| IBIS file stm32mp211_213_215_vfbga273.ibs
[IBIS ver] 5.1
[File name] stm32mp211_213_215_vfbga273.ibs
[File Rev] 0.4
[Date] 09-10-2025
[Source] Data Created at STMicroelectronics
[Notes]  File originated from ELDO simulations.
[Disclaimer]  This information is for modeling purpose only and is
   not guaranted. The information is subject to change without
   notice.
[Copyright] Copyright 2025 STMicroelectronics Inc.
|   Component stm32mp211_213_215_vfbga273
[Component] stm32mp211_213_215_vfbga273
[Manufacturer] STMicroelectronics
[Package]
| variable   typ   min   max
R_pkg  0  NA  NA
L_pkg  0  NA  NA
C_pkg  0  NA  NA
[Pin]   signal_name   model_name
1A1  VSS  gnd
1A3  VSS  gnd
1A5  VSS  gnd
1A7  VSS  gnd
1B2  VSS  gnd
1B4  VSS  gnd
1B6  VDDCPU  nc
1B8  VSS  gnd
1C1  VDDCORE  nc
1C3  VDDCORE  nc
1C5  VDDCPU  nc
1C7  VDDCPU  nc
1D2  VDDCORE  nc
1D4  VDDCORE  nc
1D6  VDDCPU  nc
1D8  VDDCPU  nc
1E1  VSS  gnd
1E3  VSS  gnd
1E5  VSS  gnd
1E7  VSS  gnd
1F2  VSS  gnd
1F4  VSS  gnd
1F6  VSS  gnd
1F8  VSS  gnd
1G1  VDD  power
1G3  VDD  power
1G5  VDDCORE  nc
1G7  VSS  gnd
1H2  VDD  power
1H4  VDD  power
1H6  VDDCORE  nc
1H8  VDDCORE  nc
A1  VSS  gnd
A2  CSI_D1P  DPHY_IBIS_L1
A3  CSI_CKP  DPHY_IBIS_L1
A6  PD3  io8_tt
A7  PD15  io8_tt_i3c
A10  PB1  io8_tt
A11  PE0  io8_tt
A14  PE13  io8_tt
A15  PE12  io8_tt
A18  PB12  io8_tt
A19  PD13  io8_tt
A20  DDR_DQ11  mal4drv27_PAD
A21  VSS  gnd
AA1  VSS  gnd
AA2  OSC_OUT  isudq_v18
AA3  BOOT2  isudq_tt
AA6  PF10  io8_tt
AA7  PF9  io8_tt
AA10  PA14  io8_tt
AA11  PF2  io8_tt_i3c
AA14  PH12  io8_tt
AA15  PH7  io8_tt
AA18  PH4  io8_tt
AA19  USBH_HS_DM  USB2_HS_IBIS
AA20  OTG_TXRTUNE  nc
AA21  VSS  gnd
B1  CSI_D0P  DPHY_IBIS_L1
B2  CSI_D1N  DPHY_IBIS_L1
B3  CSI_CKN  DPHY_IBIS_L1
B4  PD10  io8_tt_i3c
B6  PD4  io8_tt
B7  PD8  io8_tt
B8  PB9  io8_tt
B10  PB3  io8_tt
B11  PD6  io8_tt
B12  PE2  io8_tt
B14  PE11  io8_tt
B15  PE9  io8_tt
B16  PB14  io8_tt
B18  PD12  io8_tt
B19  DDR_DQ10  mal4drv27_PAD
B20  DDR_DQ9  mal4drv27_PAD
B21  DDR_DQ8  mal4drv27_PAD
C1  CSI_D0N  DPHY_IBIS_L1
C2  VDDCSI  nc
C3  CSI_REXT  nc
C4  PD2  io8_tt
C5  PB7  io8_tt
C6  PB11  io8_tt
C7  PD1  io8_tt
C8  PB10  io8_tt
C9  PD9  io8_tt
C10  PD5  io8_tt
C11  PE1  io8_tt
C12  PE3  io8_tt
C13  PE8  io8_tt
C14  PE7  io8_tt
C15  PE10  io8_tt
C16  PB13  io8_tt
C17  PD14  io8_tt
C18  DDR_RESETN  nc
C19  DDR_DQ15  mal4drv27_PAD
C20  DDR_DQS1N  mal4drv27_PAD
C21  DDR_DQS1P  mal4drv27_PAD
D2  VDDA18CSI  power
D3  PI6  io8_tt
D4  PD11  io8_tt_i3c
D6  PB6  io8_tt
D8  PD0  io8_tt
D10  PE5  io8_tt
D12  PE4  io8_tt
D14  PE14  io8_tt
D16  VDDA18PLL1  nc
D18  DDR_A9  mal4drv20_PAD
D19  DDR_DQ14  mal4drv27_PAD
D20  DDR_DQM1  mal4drv27_PAD
E3  PG2  io8_tt_i3c
E4  PC5  io8_tt_i3c
E5  PI5  io8_tt
E7  PB5  io8_tt_i3c
E9  PB2  io8_tt
E11  PE15  io8_tt
E13  PE6  io8_tt
E15  PD7  io8_tt
E17  DDR_A3  mal4drv20_PAD
E19  DDR_DQ12  mal4drv27_PAD
F1  PI1  io8_tt_i3c
F2  PA7  io8_tt
F3  PF5  io8_tt
F4  PI0  io8_tt
F6  VSS  gnd
F8  VDDIO3  power
F10  VDDIO3  power
F12  VDDIO2  power
F14  VDDIO1  power
F16  VDDA18DDR  nc
F18  DDR_A20  mal4drv20_PAD
F19  DDR_DQ13  mal4drv27_PAD
F20  DDR_A11  mal4drv20_PAD
F21  DDR_A21  mal4drv20_PAD
G1  PG14  io8_tt
G2  PG15  io8_tt
G3  PF6  io8_tt
G5  PI4  io8_tt
G17  DDR_A0  mal4drv20_PAD
G19  DDR_A1  mal4drv20_PAD
G20  DDR_A10  mal4drv20_PAD
G21  DDR_A22  mal4drv20_PAD
H2  PG12  io8_tt
H3  PG11  io8_tt
H4  PG10  io8_tt
H6  V08CAP  nc
H16  VDDQDDR  power
H18  DDR_A25  mal4drv20_PAD
H19  DDR_A8  mal4drv20_PAD
H20  DDR_A23  mal4drv20_PAD
J3  PG9  io8_tt
J5  PC0  io8_tt
J17  DDR_A18  mal4drv20_PAD
J19  DDR_A2  mal4drv20_PAD
K1  PA5  io8_tt
K2  PH5  io8_tt
K3  PG8  io8_tt
K4  PZ0  io8_tt_i3c_tamp
K6  PZ3  io8_tt_i3c_tamp
K16  VDDQDDR  power
K18  DDR_A31  mal4drv20_PAD
K19  DDR_A14  mal4drv20_PAD
K20  DDR_A26  mal4drv20_PAD
K21  DDR_A13  mal4drv20_PAD
L1  VDDA18AON  power
L2  VSSAON  nc
L3  PG7  io8_tt
L5  PZ1  io8_tt_i3c_tamp
L17  DDR_A12  mal4drv20_PAD
L19  DDR_A27  mal4drv20_PAD
L20  DDR_A5  mal4drv20_PAD
L21  DDR_A4  mal4drv20_PAD
M2  PA10  io8_tt
M3  PF4  io8_tt
M4  PG5  io8_tt
M6  VBAT  power
M16  VDDQDDR  power
M18  DDR_A6  mal4drv20_PAD
M19  DDR_A28  mal4drv20_PAD
M20  DDR_A15  mal4drv20_PAD
N3  PB15  io8_tt
N5  PA1  io8_tt_i3c
N17  DDR_ZQ  nc
N19  DDR_A16  mal4drv20_PAD
P1  PF13  io8_tt
P2  PF15  io8_tt
P3  PC11  io8_tt
P4  PF7  io8_tt
P6  PG4  io8_tt
P16  VDDQDDR  power
P18  DDR_A7  mal4drv20_PAD
P19  DDR_A29  mal4drv20_PAD
P20  DDR_A17  mal4drv20_PAD
P21  DDR_A30  mal4drv20_PAD
R1  OSC32_IN  isudq_v18
R2  OSC32_OUT  isudq_v18
R3  PDR_ON  nc
R5  PC4  io8_tt
R17  VDDA18PLL2  nc
R19  DDR_DQ6  mal4drv27_PAD
R20  DDR_DQ4  mal4drv27_PAD
R21  DDR_DQ5  mal4drv27_PAD
T2  NRSTC1MS  io8_tt
T3  PG13  io8_tt_i3c
T4  PC13  io8_tt
T6  VSSA  nc
T8  PG0  io8_tt_i3c
T10  PC7  io8_tt
T12  PC3  io8_tt
T14  PF8  io8_tt
T16  PA9  io8_tt
T18  DDR_VREF  nc
T19  DDR_DQS0P  mal4drv27_PAD
T20  DDR_DQ7  mal4drv27_PAD
U3  PF12  io8_tt
U5  PI8  io8_tt
U7  PG1  io8_tt_i3c
U9  PC10  io8_tt
U11  PA15  io8_tt_i3c
U13  PF3  io8_tt
U15  PH9  io8_tt
U17  DDR_DQM0  mal4drv27_PAD
U19  DDR_DQS0N  mal4drv27_PAD
V1  JTCK_SWCLK  io8_tt
V2  JTMS_SWDIO  io8_tt
V3  NJTRST  io8_tt
V4  PWR_CPUON  io8_tt
V6  PG3  io8_tt
V8  ANA0  nc
V10  PC1  io8_tt_i3c
V12  PA13  io8_tt
V14  PH10  io8_tt
V16  PA8  io8_tt_i3c
V18  VDDA18USB  power
V19  DDR_DQ1  mal4drv27_PAD
V20  DDR_DQ0  mal4drv27_PAD
V21  DDR_DQ2  mal4drv27_PAD
W1  JTDO_TRACESWO  io8_tt
W2  JTDI  io8_tt
W3  PWR_LP  io8_tt
W4  PWR_ON  io8_tt
W5  BOOT3  isudq_tt
W6  VDDA18ADC  power
W7  PF11  io8_tt
W8  VREFN  nc
W9  ANA1  nc
W10  PC9  io8_tt
W11  PF1  io8_tt
W12  PC6  io8_tt_i3c
W13  PH13  io8_tt
W14  PH11  io8_tt
W15  PA11  io8_tt
W16  PA6  io8_tt
W17  PA2  io8_tt_i3c
W18  VSS  gnd
W19  VDD33USB  power
W20  USBH_HS_TXRTUNE  nc
W21  DDR_DQ3  mal4drv27_PAD
Y1  NRST  nc
Y2  OSC_IN  isudq_v18
Y3  BOOT1  isudq_tt
Y4  BOOT0  isudq_tt
Y6  PA0  io8_tt
Y7  PC12  io8_tt_i3c
Y8  VREFP  nc
Y10  PC8  io8_tt
Y11  PF0  io8_tt_i3c
Y12  PC2  io8_tt
Y14  PA12  io8_tt_i3c
Y15  PH8  io8_tt
Y16  PA4  io8_tt
Y18  PA3  io8_tt_i3c
Y19  USBH_HS_DP  USB2_HS_IBIS
Y20  OTG_HSDP  USB2_HS_IBIS
Y21  OTG_HSDM  USB2_HS_IBIS
[Package Model]   503-fcvfbga-11x11-273-240814
[Pin Mapping]   pulldown_ref   pullup_ref   | Comment
1A1  gnd  nc
1A3  gnd  nc
1A5  gnd  nc
1A7  gnd  nc
1B2  gnd  nc
1B4  gnd  nc
1B6  nc  nc
1B8  gnd  nc
1C1  nc  nc
1C3  nc  nc
1C5  nc  nc
1C7  nc  nc
1D2  nc  nc
1D4  nc  nc
1D6  nc  nc
1D8  nc  nc
1E1  gnd  nc
1E3  gnd  nc
1E5  gnd  nc
1E7  gnd  nc
1F2  gnd  nc
1F4  gnd  nc
1F6  gnd  nc
1F8  gnd  nc
1G1  nc  vdd
1G3  nc  vdd
1G5  nc  nc
1G7  gnd  nc
1H2  nc  vdd
1H4  nc  vdd
1H6  nc  nc
1H8  nc  nc
A1  gnd  nc
A2  gnd  VDDA18CSI
A3  gnd  VDDA18CSI
A6  gnd  vddio3
A7  gnd  vdd
A10  gnd  vdd
A11  gnd  vddio1
A14  gnd  vddio2
A15  gnd  vddio2
A18  gnd  vdd
A19  gnd  vdd
A20  gnd  vddqddr
A21  gnd  nc
AA1  gnd  nc
AA2  gnd  vdda18aon
AA3  gnd  vdd
AA6  gnd  vdd
AA7  gnd  vdd
AA10  gnd  vdd
AA11  gnd  vdd
AA14  gnd  vdd
AA15  gnd  vdd
AA18  gnd  vdd
AA19  gnd  VDD33USB
AA20  nc  nc
AA21  gnd  nc
B1  gnd  VDDA18CSI
B2  gnd  VDDA18CSI
B3  gnd  VDDA18CSI
B4  gnd  vddio3
B6  gnd  vddio3
B7  gnd  vddio3
B8  gnd  vdd
B10  gnd  vdd
B11  gnd  vddio3
B12  gnd  vddio1
B14  gnd  vddio2
B15  gnd  vddio1
B16  gnd  vdd
B18  gnd  vdd
B19  gnd  vddqddr
B20  gnd  vddqddr
B21  gnd  vddqddr
C1  gnd  VDDA18CSI
C2  nc  nc
C3  nc  nc
C4  gnd  vddio3
C5  gnd  vdd
C6  gnd  vdd
C7  gnd  vddio3
C8  gnd  vdd
C9  gnd  vddio3
C10  gnd  vddio3
C11  gnd  vddio1
C12  gnd  vddio1
C13  gnd  vddio1
C14  gnd  vddio1
C15  gnd  vddio2
C16  gnd  vdd
C17  gnd  vdd
C18  nc  nc
C19  gnd  vddqddr
C20  gnd  vddqddr
C21  gnd  vddqddr
D2  nc  VDDA18CSI
D3  gnd  vdd
D4  gnd  vddio3
D6  gnd  vdd
D8  gnd  vddio3
D10  gnd  vddio1
D12  gnd  vddio1
D14  gnd  vddio2
D16  nc  nc
D18  gnd  vddqddr
D19  gnd  vddqddr
D20  gnd  vddqddr
E3  gnd  vdd
E4  gnd  vdd
E5  gnd  vdd
E7  gnd  vdd
E9  gnd  vdd
E11  gnd  vddio2
E13  gnd  vddio1
E15  gnd  vddio3
E17  gnd  vddqddr
E19  gnd  vddqddr
F1  gnd  vdd
F2  gnd  vdd
F3  gnd  vdd
F4  gnd  vdd
F6  gnd  nc
F8  nc  vddio3
F10  nc  vddio3
F12  nc  vddio2
F14  nc  vddio1
F16  nc  nc
F18  gnd  vddqddr
F19  gnd  vddqddr
F20  gnd  vddqddr
F21  gnd  vddqddr
G1  gnd  vdd
G2  gnd  vdd
G3  gnd  vdd
G5  gnd  vdd
G17  gnd  vddqddr
G19  gnd  vddqddr
G20  gnd  vddqddr
G21  gnd  vddqddr
H2  gnd  vdd
H3  gnd  vdd
H4  gnd  vdd
H6  nc  nc
H16  nc  vddqddr
H18  gnd  vddqddr
H19  gnd  vddqddr
H20  gnd  vddqddr
J3  gnd  vdd
J5  gnd  vdd
J17  gnd  vddqddr
J19  gnd  vddqddr
K1  gnd  vdd
K2  gnd  vdd
K3  gnd  vdd
K4  gnd  vdd  | Depending on IO usage
| K4  gnd  vsw  | Depending on IO usage
K6  gnd  vdd  | Depending on IO usage
| K6  gnd  vsw  | Depending on IO usage
K16  nc  vddqddr
K18  gnd  vddqddr
K19  gnd  vddqddr
K20  gnd  vddqddr
K21  gnd  vddqddr
L1  nc  vdda18aon
L2  nc  nc
L3  gnd  vdd
L5  gnd  vdd  | Depending on IO usage
| L5  gnd  vsw  | Depending on IO usage
L17  gnd  vddqddr
L19  gnd  vddqddr
L20  gnd  vddqddr
L21  gnd  vddqddr
M2  gnd  vdd
M3  gnd  vdd
M4  gnd  vdd
M6  nc  vsw
M16  nc  vddqddr
M18  gnd  vddqddr
M19  gnd  vddqddr
M20  gnd  vddqddr
N3  gnd  vdd
N5  gnd  vdd
N17  nc  nc
N19  gnd  vddqddr
P1  gnd  vdd
P2  gnd  vdd
P3  gnd  vdd
P4  gnd  vdd
P6  gnd  vdd
P16  nc  vddqddr
P18  gnd  vddqddr
P19  gnd  vddqddr
P20  gnd  vddqddr
P21  gnd  vddqddr
R1  gnd  vdd  | Depending on IO usage
| R1  gnd  vsw  | Depending on IO usage
R2  gnd  vdd  | Depending on IO usage
| R2  gnd  vsw  | Depending on IO usage
R3  nc  nc
R5  gnd  vdd
R17  nc  nc
R19  gnd  vddqddr
R20  gnd  vddqddr
R21  gnd  vddqddr
T2  gnd  vdd
T3  gnd  vdd
T4  gnd  vdd  | Depending on IO usage
| T4  gnd  vsw  | Depending on IO usage
T6  nc  nc
T8  gnd  vdd
T10  gnd  vdd
T12  gnd  vdd
T14  gnd  vdd
T16  gnd  vdd
T18  nc  nc
T19  gnd  vddqddr
T20  gnd  vddqddr
U3  gnd  vdd
U5  gnd  vdd
U7  gnd  vdd
U9  gnd  vdd
U11  gnd  vdd
U13  gnd  vdd
U15  gnd  vdd
U17  gnd  vddqddr
U19  gnd  vddqddr
V1  gnd  vdd
V2  gnd  vdd
V3  gnd  vdd
V4  gnd  vdd
V6  gnd  vdd
V8  nc  nc
V10  gnd  vdd
V12  gnd  vdd
V14  gnd  vdd
V16  gnd  vdd
V18  nc  vdda18usb
V19  gnd  vddqddr
V20  gnd  vddqddr
V21  gnd  vddqddr
W1  gnd  vdd
W2  gnd  vdd
W3  gnd  vdd
W4  gnd  vdd
W5  gnd  vdd
W6  nc  vdda18adc
W7  gnd  vdd
W8  nc  nc
W9  nc  nc
W10  gnd  vdd
W11  gnd  vdd
W12  gnd  vdd
W13  gnd  vdd
W14  gnd  vdd
W15  gnd  vdd
W16  gnd  vdd
W17  gnd  vdd
W18  gnd  nc
W19  nc  VDD33USB
W20  nc  nc
W21  gnd  vddqddr
Y1  nc  nc
Y2  gnd  vdda18aon
Y3  gnd  vdd
Y4  gnd  vdd
Y6  gnd  vdd
Y7  gnd  vdd
Y8  nc  nc
Y10  gnd  vdd
Y11  gnd  vdd
Y12  gnd  vdd
Y14  gnd  vdd
Y15  gnd  vdd
Y16  gnd  vdd
Y18  gnd  vdd
Y19  gnd  VDD33USB
Y20  gnd  VDD33USB
Y21  gnd  VDD33USB
[Diff Pin]  inv_pin  vdiff  tdelay_typ  tdelay_min  tdelay_max
B3  A3  NA  NA  NA  NA
C1  B1  NA  NA  NA  NA
B2  A2  NA  NA  NA  NA
T19  U19  NA  NA  NA  NA
C21  C20  NA  NA  NA  NA
Y19  AA19  NA  NA  NA  NA   |USBH_HS_DP _DM
Y20  Y21  NA  NA  NA  NA   |USBH_HS_DP _DM
L21  L20  NA  NA  NA  NA
[Model Selector] USB2_HS_IBIS
USB2_HSRX   USB2 HSRX model
USB2_HSTX_00_0_01_0011_11   TuningBits_AMP_PULSE_RISE_REF_XV=00_0_01_0011_11
USB2_HSTX_00_0_10_0101_11   TuningBits_AMP_PULSE_RISE_REF_XV=00_0_10_0101_11
USB2_HSTX_00_0_11_0111_11   TuningBits_AMP_PULSE_RISE_REF_XV=00_0_11_0111_11
USB2_HSTX_00_1_01_0011_11   TuningBits_AMP_PULSE_RISE_REF_XV=00_1_01_0011_11
USB2_HSTX_00_1_10_0101_11   TuningBits_AMP_PULSE_RISE_REF_XV=00_1_10_0101_11
USB2_HSTX_00_1_11_0111_11   TuningBits_AMP_PULSE_RISE_REF_XV=00_1_11_0111_11
USB2_HSTX_01_0_01_0011_11   TuningBits_AMP_PULSE_RISE_REF_XV=01_0_01_0011_11
USB2_HSTX_01_0_10_0101_11   TuningBits_AMP_PULSE_RISE_REF_XV=01_0_10_0101_11
USB2_HSTX_01_0_11_0111_11   TuningBits_AMP_PULSE_RISE_REF_XV=01_0_11_0111_11
USB2_HSTX_01_1_01_0011_11   TuningBits_AMP_PULSE_RISE_REF_XV=01_1_01_0011_11
USB2_HSTX_01_1_10_0101_11   TuningBits_AMP_PULSE_RISE_REF_XV=01_1_10_0101_11
USB2_HSTX_01_1_11_0111_11   TuningBits_AMP_PULSE_RISE_REF_XV=01_1_11_0111_11
USB2_HSTX_10_0_01_0011_11   TuningBits_AMP_PULSE_RISE_REF_XV=10_0_01_0011_11
USB2_HSTX_10_0_10_0101_11   TuningBits_AMP_PULSE_RISE_REF_XV=10_0_10_0101_11
USB2_HSTX_10_0_11_0111_11   TuningBits_AMP_PULSE_RISE_REF_XV=10_0_11_0111_11
USB2_HSTX_10_1_01_0011_11   TuningBits_AMP_PULSE_RISE_REF_XV=10_1_01_0011_11
USB2_HSTX_10_1_10_0101_11   TuningBits_AMP_PULSE_RISE_REF_XV=10_1_10_0101_11
USB2_HSTX_10_1_11_0111_11   TuningBits_AMP_PULSE_RISE_REF_XV=10_1_11_0111_11
[Model Selector] DPHY_IBIS_L1
DPHY_RX_2P5G_L1   DPHY HSRX model at 2.5Gbps for lane 1
DPHY_RX_1P5G_L1   DPHY HSRX model at 1.5Gbps for lane 1
[Model Selector] io8_tt
io8_tt_ls_3v3 "GPIO - 3V tolerant - low speed - 3.3V range"
io8_tt_ms_3v3 "GPIO - 3V tolerant - med speed - 3.3V range"
io8_tt_fs_3v3 "GPIO - 3V tolerant - fast speed - 3.3V range"
io8_tt_hs_3v3 "GPIO - 3V tolerant - high speed - 3.3V range"
io8_tt_hslv_ls_1v8 "GPIO low voltage optimization - 3V tolerant - low speed - 1.8V range"
io8_tt_hslv_ms_1v8 "GPIO low voltage optimization - 3V tolerant - med speed - 1.8V range"
io8_tt_hslv_fs_1v8 "GPIO low voltage optimization - 3V tolerant - fast speed - 1.8V range"
io8_tt_hslv_hs_1v8 "GPIO low voltage optimization - 3V tolerant - high speed - 1.8V range"
[Model Selector] io8_tt_i3c
io8_tt_ls_3v3 "GPIO - 3V tolerant - low speed - 3.3V range"
io8_tt_ms_3v3 "GPIO - 3V tolerant - med speed - 3.3V range"
io8_tt_fs_3v3 "GPIO - 3V tolerant - fast speed - 3.3V range"
io8_tt_hs_3v3 "GPIO - 3V tolerant - high speed - 3.3V range"
io8_tt_hslv_ls_1v8 "GPIO low voltage optimization - 3V tolerant - low speed - 1.8V range"
io8_tt_hslv_ms_1v8 "GPIO low voltage optimization - 3V tolerant - med speed - 1.8V range"
io8_tt_hslv_fs_1v8 "GPIO low voltage optimization - 3V tolerant - fast speed - 1.8V range"
io8_tt_hslv_hs_1v8 "GPIO low voltage optimization - 3V tolerant - high speed - 1.8V range"
io8_tt_i3c_ls_3v3 "GPIO with I3C open-drain - 3V tolerant - low speed - 3.3V range"
io8_tt_i3c_ms_3v3 "GPIO with I3C open-drain - 3V tolerant - med speed - 3.3V range"
io8_tt_i3c_fs_3v3 "GPIO with I3C open-drain - 3V tolerant - fast speed - 3.3V range"
io8_tt_i3c_hs_3v3 "GPIO with I3C open-drain - 3V tolerant - high speed - 3.3V range"
io8_tt_hslv_i3c_ls_1v8 "GPIO low voltage optimization with I3C open-drain - 3V tolerant - low speed - 1.8V range"
io8_tt_hslv_i3c_ms_1v8 "GPIO low voltage optimization with I3C open-drain - 3V tolerant - med speed - 1.8V range"
io8_tt_hslv_i3c_fs_1v8 "GPIO low voltage optimization with I3C open-drain - 3V tolerant - fast speed - 1.8V range"
io8_tt_hslv_i3c_hs_1v8 "GPIO low voltage optimization with I3C open-drain - 3V tolerant - high speed - 1.8V range"
io8_tt_i3c_fmp_3v3 "GPIO with I3C fm+ open-drain - 3V tolerant - 3.3V range"
[Model Selector] io8_tt_i3c_tamp
io8_tt_ls_3v3 "GPIO - 3V tolerant - low speed - 3.3V range"
io8_tt_ms_3v3 "GPIO - 3V tolerant - med speed - 3.3V range"
io8_tt_fs_3v3 "GPIO - 3V tolerant - fast speed - 3.3V range"
io8_tt_hs_3v3 "GPIO - 3V tolerant - high speed - 3.3V range"
io8_tt_hslv_ls_1v8 "GPIO low voltage optimization - 3V tolerant - low speed - 1.8V range"
io8_tt_hslv_ms_1v8 "GPIO low voltage optimization - 3V tolerant - med speed - 1.8V range"
io8_tt_hslv_fs_1v8 "GPIO low voltage optimization - 3V tolerant - fast speed - 1.8V range"
io8_tt_hslv_hs_1v8 "GPIO low voltage optimization - 3V tolerant - high speed - 1.8V range"
io8_tt_i3c_ls_3v3 "GPIO with I3C open-drain - 3V tolerant - low speed - 3.3V range"
io8_tt_i3c_ms_3v3 "GPIO with I3C open-drain - 3V tolerant - med speed - 3.3V range"
io8_tt_i3c_fs_3v3 "GPIO with I3C open-drain - 3V tolerant - fast speed - 3.3V range"
io8_tt_i3c_hs_3v3 "GPIO with I3C open-drain - 3V tolerant - high speed - 3.3V range"
io8_tt_hslv_i3c_ls_1v8 "GPIO low voltage optimization with I3C open-drain - 3V tolerant - low speed - 1.8V range"
io8_tt_hslv_i3c_ms_1v8 "GPIO low voltage optimization with I3C open-drain - 3V tolerant - med speed - 1.8V range"
io8_tt_hslv_i3c_fs_1v8 "GPIO low voltage optimization with I3C open-drain - 3V tolerant - fast speed - 1.8V range"
io8_tt_hslv_i3c_hs_1v8 "GPIO low voltage optimization with I3C open-drain - 3V tolerant - high speed - 1.8V range"
io8_tt_i3c_fmp_3v3 "GPIO with I3C fm+ open-drain - 3V tolerant - 3.3V range"
io8_tt_tamp_3v3 "IO tamper - 3V tolerant - 3.3V range"
io8_tt_tamp_1v8 "IO tamper - 3V tolerant - 1.8V range"
[Model Selector] isudq_tt
isudq_tt_3v3 "Input Buffer - 3V tolerant - 3.3V range"
isudq_tt_1v8 "Input Buffer - 3V tolerant - 1.8V range"
|[Model Selector] isudq_v18
|isudq_v18_1v8 "Input Buffer - 1.8V range "
[Model Selector]   mal4drv20_PAD
mal4drv20_d3l_40   DDR3L mal4drv20 cell  Z0=40-Ohm Driver
mal4drv20_d3l_60   DDR3L mal4drv20 cell  Z0=60-Ohm Driver
mal4drv20_d3l_120   DDR3L mal4drv20 cell  Z0=120-Ohm Driver
mal4drv20_d3_20   DDR3 mal4drv20 cell  Z0=20-Ohm Driver
mal4drv20_d3_24   DDR3 mal4drv20 cell  Z0=24-Ohm Driver
mal4drv20_d3_30   DDR3 mal4drv20 cell  Z0=30-Ohm Driver
mal4drv20_d3_40   DDR3 mal4drv20 cell  Z0=40-Ohm Driver
mal4drv20_d3_60   DDR3 mal4drv20 cell  Z0=60-Ohm Driver
mal4drv20_d4_20   DDR4 mal4drv20 cell  Z0=20-Ohm Driver
mal4drv20_d4_24   DDR4 mal4drv20 cell  Z0=24-Ohm Driver
mal4drv20_d4_30   DDR4 mal4drv20 cell  Z0=30-Ohm Driver
mal4drv20_d4_40   DDR4 mal4drv20 cell  Z0=40-Ohm Driver
mal4drv20_d4_60   DDR4 mal4drv20 cell  Z0=60-Ohm Driver
mal4drv20_dl4_20   LPDDR4 mal4drv20 cell  Z0=20-Ohm Driver
mal4drv20_dl4_24   LPDDR4 mal4drv20 cell  Z0=24-Ohm Driver
mal4drv20_dl4_30   LPDDR4 mal4drv20 cell  Z0=30-Ohm Driver
mal4drv20_dl4_40   LPDDR4 mal4drv20 cell  Z0=40-Ohm Driver
mal4drv20_dl4_60   LPDDR4 mal4drv20 cell  Z0=60-Ohm Driver
[Model Selector]   mal4drv27_PAD
mal4drv27_d3l_40   DDR3L mal4drv27 cell  Z0=40-Ohm Driver
mal4drv27_d3l_48   DDR3L mal4drv27 cell  Z0=48-Ohm Driver
mal4drv27_d3l_60   DDR3L mal4drv27 cell  Z0=60-Ohm Driver
mal4drv27_d3l_80   DDR3L mal4drv27 cell  Z0=80-Ohm Driver
mal4drv27_d3l_120   DDR3L mal4drv27 cell  Z0=120-Ohm Driver
mal4drv27_d3l_240   DDR3L mal4drv27 cell  Z0=240-Ohm Driver
mal4drv27_d3l_odt120   DDR3L mal4drv27 cell 120-Ohm ODT Receiver
mal4drv27_d3l_odt60   DDR3L mal4drv27 cell 60-Ohm ODT Receiver
mal4drv27_d3l_odtoff   DDR3L mal4drv27 cell ODT OFF Receiver
mal4drv27_d3_28   DDR3 mal4drv27 cell  Z0=28-Ohm Driver
mal4drv27_d3_34   DDR3 mal4drv27 cell  Z0=34-Ohm Driver
mal4drv27_d3_40   DDR3 mal4drv27 cell  Z0=40-Ohm Driver
mal4drv27_d3_53   DDR3 mal4drv27 cell  Z0=53-Ohm Driver
mal4drv27_d3_odt120   DDR3 mal4drv27 cell 120-Ohm ODT Receiver
mal4drv27_d3_odt60   DDR3 mal4drv27 cell 60-Ohm ODT Receiver
mal4drv27_d4_28   DDR4 mal4drv27 cell  Z0=28-Ohm Driver
mal4drv27_d4_34   DDR4 mal4drv27 cell  Z0=34-Ohm Driver
mal4drv27_d4_40   DDR4 mal4drv27 cell  Z0=40-Ohm Driver
mal4drv27_d4_53   DDR4 mal4drv27 cell  Z0=53-Ohm Driver
mal4drv27_d4_odt120   DDR4 mal4drv27 cell 120-Ohm ODT Receiver
mal4drv27_d4_odt240   DDR4 mal4drv27 cell 240-Ohm ODT Receiver
mal4drv27_d4_odt48   DDR4 mal4drv27 cell 48-Ohm ODT Receiver
mal4drv27_d4_odt60   DDR4 mal4drv27 cell 60-Ohm ODT Receiver
mal4drv27_d4_odt80   DDR4 mal4drv27 cell 80-Ohm ODT Receiver
mal4drv27_dl4_28   LPDDR4 mal4drv27 cell  Z0=28-Ohm Driver
mal4drv27_dl4_34   LPDDR4 mal4drv27 cell  Z0=34-Ohm Driver
mal4drv27_dl4_40   LPDDR4 mal4drv27 cell  Z0=40-Ohm Driver
mal4drv27_dl4_53   LPDDR4 mal4drv27 cell  Z0=53-Ohm Driver
mal4drv27_dl4_odt48   LPDDR4 mal4drv27 cell 48-Ohm ODT Receiver
mal4drv27_dl4_odt60   LPDDR4 mal4drv27 cell 60-Ohm ODT Receiver
[Define Package Model]  503-fcvfbga-11x11-273-240814
[Manufacturer]  unknown
[OEM]  unknown
[Description]  unknown
[Number Of Pins]  235
[Pin Numbers]
| Pin Name Terminal   Net Name   Starting Node   Ending Node
V8 | ANA0
W9 | ANA1
Y4 | BOOT0
Y3 | BOOT1
AA3 | BOOT2
W5 | BOOT3
B3 | CSI_CKN
A3 | CSI_CKP
C1 | CSI_D0N
B1 | CSI_D0P
B2 | CSI_D1N
A2 | CSI_D1P
C3 | CSI_REXT
G17 | DDR_A0
G19 | DDR_A1
J19 | DDR_A2
E17 | DDR_A3
L21 | DDR_A4
L20 | DDR_A5
M18 | DDR_A6
P18 | DDR_A7
H19 | DDR_A8
D18 | DDR_A9
G20 | DDR_A10
F20 | DDR_A11
L17 | DDR_A12
K21 | DDR_A13
K19 | DDR_A14
M20 | DDR_A15
N19 | DDR_A16
P20 | DDR_A17
J17 | DDR_A18
F18 | DDR_A20
F21 | DDR_A21
G21 | DDR_A22
H20 | DDR_A23
H18 | DDR_A25
K20 | DDR_A26
L19 | DDR_A27
M19 | DDR_A28
P19 | DDR_A29
P21 | DDR_A30
K18 | DDR_A31
V20 | DDR_DQ0
V19 | DDR_DQ1
V21 | DDR_DQ2
W21 | DDR_DQ3
R20 | DDR_DQ4
R21 | DDR_DQ5
R19 | DDR_DQ6
T20 | DDR_DQ7
B21 | DDR_DQ8
B20 | DDR_DQ9
B19 | DDR_DQ10
A20 | DDR_DQ11
E19 | DDR_DQ12
F19 | DDR_DQ13
D19 | DDR_DQ14
C19 | DDR_DQ15
U17 | DDR_DQM0
D20 | DDR_DQM1
U19 | DDR_DQS0N
T19 | DDR_DQS0P
C20 | DDR_DQS1N
C21 | DDR_DQS1P
C18 | DDR_RESETN
T18 | DDR_VREF
N17 | DDR_ZQ
V1 | JTCK_SWCLK
W2 | JTDI
W1 | JTDO_TRACESWO
V2 | JTMS_SWDIO
V3 | NJTRST
Y1 | NRST
T2 | NRSTC1MS
R1 | OSC32_IN
R2 | OSC32_OUT
Y2 | OSC_IN
AA2 | OSC_OUT
Y21 | OTG_HSDM
Y20 | OTG_HSDP
AA20 | OTG_TXRTUNE
Y6 | PA0
N5 | PA1
W17 | PA2
Y18 | PA3
Y16 | PA4
K1 | PA5
W16 | PA6
F2 | PA7
V16 | PA8
T16 | PA9
M2 | PA10
W15 | PA11
Y14 | PA12
V12 | PA13
AA10 | PA14
U11 | PA15
A10 | PB1
E9 | PB2
B10 | PB3
E7 | PB5
D6 | PB6
C5 | PB7
B8 | PB9
C8 | PB10
C6 | PB11
A18 | PB12
C16 | PB13
B16 | PB14
N3 | PB15
J5 | PC0
V10 | PC1
Y12 | PC2
T12 | PC3
R5 | PC4
E4 | PC5
W12 | PC6
T10 | PC7
Y10 | PC8
W10 | PC9
U9 | PC10
P3 | PC11
Y7 | PC12
T4 | PC13
D8 | PD0
C7 | PD1
C4 | PD2
A6 | PD3
B6 | PD4
C10 | PD5
B11 | PD6
E15 | PD7
B7 | PD8
C9 | PD9
B4 | PD10
D4 | PD11
B18 | PD12
A19 | PD13
C17 | PD14
A7 | PD15
R3 | PDR_ON
A11 | PE0
C11 | PE1
B12 | PE2
C12 | PE3
D12 | PE4
D10 | PE5
E13 | PE6
C14 | PE7
C13 | PE8
B15 | PE9
C15 | PE10
B14 | PE11
A15 | PE12
A14 | PE13
D14 | PE14
E11 | PE15
Y11 | PF0
W11 | PF1
AA11 | PF2
U13 | PF3
M3 | PF4
F3 | PF5
G3 | PF6
P4 | PF7
T14 | PF8
AA7 | PF9
AA6 | PF10
W7 | PF11
U3 | PF12
P1 | PF13
P2 | PF15
T8 | PG0
U7 | PG1
E3 | PG2
V6 | PG3
P6 | PG4
M4 | PG5
L3 | PG7
K3 | PG8
J3 | PG9
H4 | PG10
H3 | PG11
H2 | PG12
T3 | PG13
G1 | PG14
G2 | PG15
AA18 | PH4
K2 | PH5
AA15 | PH7
Y15 | PH8
U15 | PH9
V14 | PH10
W14 | PH11
AA14 | PH12
W13 | PH13
F4 | PI0
F1 | PI1
G5 | PI4
E5 | PI5
D3 | PI6
U5 | PI8
V4 | PWR_CPUON
W3 | PWR_LP
W4 | PWR_ON
K4 | PZ0
L5 | PZ1
K6 | PZ3
AA19 | USBH_HS_DM
Y19 | USBH_HS_DP
W20 | USBH_HS_TXRTUNE
H6 | V08CAP
M6 | VBAT
W19 | VDD33USB
1G1 | VDD
W6 | VDDA18ADC
L1 | VDDA18AON
D2 | VDDA18CSI
F16 | VDDA18DDR
D16 | VDDA18PLL1
R17 | VDDA18PLL2
V18 | VDDA18USB
1C1 | VDDCORE
1B6 | VDDCPU
C2 | VDDCSI
F14 | VDDIO1
F12 | VDDIO2
F8 | VDDIO3
H16 | VDDQDDR
Y8 | VREFP
W8 | VREFN
1A1 | VSS
T6 | VSSA
L2 | VSSAON
|[Merged Pins]  1G1
|1G3  |  VDD
|1H2  |  VDD
|1H4  |  VDD
|[Merged Pins]  1C1
|1C3  |  VDDCORE
|1D2  |  VDDCORE
|1D4  |  VDDCORE
|1G5  |  VDDCORE
|1H6  |  VDDCORE
|1H8  |  VDDCORE
|[Merged Pins]  1B6
|1C5  |  VDDCPU
|1C7  |  VDDCPU
|1D6  |  VDDCPU
|1D8  |  VDDCPU
|[Merged Pins]  F8
|F10  |  VDDIO3
|[Merged Pins]  H16
|K16  |  VDDQDDR
|M16  |  VDDQDDR
|P16  |  VDDQDDR
|[Merged Pins]  1A1
|1A3  |  VSS
|1A5  |  VSS
|1A7  |  VSS
|1B2  |  VSS
|1B4  |  VSS
|1B8  |  VSS
|1E1  |  VSS
|1E3  |  VSS
|1E5  |  VSS
|1E7  |  VSS
|1F2  |  VSS
|1F4  |  VSS
|1F6  |  VSS
|1F8  |  VSS
|1G7  |  VSS
|A1  |  VSS
|A21  |  VSS
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[Model Data]
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[End Model Data]
[End Package Model]
|End [Component]
| Models and submodels in the file (91): USB2_HSRX (Input), USB2_HSTX_00_0_01_0011_11 (Output), USB2_HSTX_00_0_10_0101_11 (Output), USB2_HSTX_00_0_11_0111_11 (Output), USB2_HSTX_00_1_01_0011_11 (Output), USB2_HSTX_00_1_10_0101_11 (Output), USB2_HSTX_00_1_11_0111_11 (Output), USB2_HSTX_01_0_01_0011_11 (Output), USB2_HSTX_01_0_10_0101_11 (Output), USB2_HSTX_01_0_11_0111_11 (Output), USB2_HSTX_01_1_01_0011_11 (Output), USB2_HSTX_01_1_10_0101_11 (Output), USB2_HSTX_01_1_11_0111_11 (Output), USB2_HSTX_10_0_01_0011_11 (Output), USB2_HSTX_10_0_10_0101_11 (Output), USB2_HSTX_10_0_11_0111_11 (Output), USB2_HSTX_10_1_01_0011_11 (Output), USB2_HSTX_10_1_10_0101_11 (Output), USB2_HSTX_10_1_11_0111_11 (Output), DPHY_RX_1P5G_L1 (Input), DPHY_RX_2P5G_L1 (Input), mal4drv20_d3_20 (I/O), mal4drv20_d3_24 (I/O), mal4drv20_d3_30 (I/O), mal4drv20_d3_40 (I/O), mal4drv20_d3_60 (I/O), mal4drv20_d4_20 (I/O), mal4drv20_d4_24 (I/O), mal4drv20_d4_30 (I/O), mal4drv20_d4_40 (I/O), mal4drv20_d4_60 (I/O), mal4drv20_dl4_20 (I/O), mal4drv20_dl4_24 (I/O), mal4drv20_dl4_30 (I/O), mal4drv20_dl4_40 (I/O), mal4drv20_dl4_60 (I/O), mal4drv27_d3_28 (I/O), mal4drv27_d3_34 (I/O), mal4drv27_d3_40 (I/O), mal4drv27_d3_53 (I/O), mal4drv27_d3_odt120 (Input), mal4drv27_d3_odt60 (Input), mal4drv27_dl4_28 (I/O), mal4drv27_dl4_34 (I/O), mal4drv27_dl4_40 (I/O), mal4drv27_dl4_53 (I/O), mal4drv27_dl4_odt48 (Input), mal4drv27_dl4_odt60 (Input), mal4drv27_d4_28 (I/O), mal4drv27_d4_34 (I/O), mal4drv27_d4_40 (I/O), mal4drv27_d4_53 (I/O), mal4drv27_d4_odt120 (Input), mal4drv27_d4_odt240 (Input), mal4drv27_d4_odt48 (Input), mal4drv27_d4_odt60 (Input), mal4drv27_d4_odt80 (Input), mal4drv20_d3l_120 (I/O), mal4drv20_d3l_40 (I/O), mal4drv20_d3l_60 (I/O), mal4drv27_d3l_120 (I/O), mal4drv27_d3l_240 (I/O), mal4drv27_d3l_40 (I/O), mal4drv27_d3l_48 (I/O), mal4drv27_d3l_60 (I/O), mal4drv27_d3l_80 (I/O), mal4drv27_d3l_odt120 (Input), mal4drv27_d3l_odt60 (Input), mal4drv27_d3l_odtoff (Input), io8_tt_fs_3v3 (I/O), io8_tt_hs_3v3 (I/O), io8_tt_hslv_fs_1v8 (I/O), io8_tt_hslv_hs_1v8 (I/O), io8_tt_hslv_i3c_fs_1v8 (I/O_open_drain), io8_tt_hslv_i3c_hs_1v8 (I/O_open_drain), io8_tt_hslv_i3c_ls_1v8 (I/O_open_drain), io8_tt_hslv_i3c_ms_1v8 (I/O_open_drain), io8_tt_hslv_ls_1v8 (I/O), io8_tt_hslv_ms_1v8 (I/O), io8_tt_i3c_fmp_3v3 (I/O_open_drain)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
